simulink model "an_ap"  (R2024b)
settings: Solver=ode45  StartTime=0.0  StopTime=50  MaxStep=.1  RelTol=1e-3  AbsTol=1e-3  EnableMultiTasking=on
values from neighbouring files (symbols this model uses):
  den = 1    [ass_appr.m]    (also in simplify.m = a(find(a):max(size(a))); ass_sis.m; ass1_sis.m; myfbode.m = b)
  den_appr = 1    [ass_appr.m]    (also in ass_sis.m)
  num = b(find(b):max(size(b)))    [simplify.m]    (also in ass_sis.m = 0; ass1_sis.m = 0; myfbode.m = a; mynyq.m = a)
  num_appr = 0    [ass_appr.m]
  T = 0; end    [ass_appr.m]    (also in ass_sis.m = 0; ass1_sis.m = 0; myfbode.m = rit)
  T_appr = 0    [ass_appr.m]    (also in ass_sis.m = 0; end)

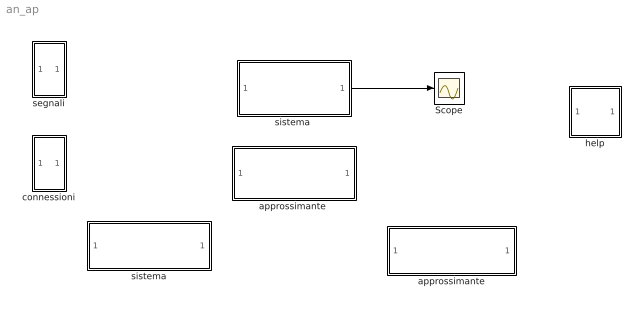
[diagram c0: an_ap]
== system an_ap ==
  Scope : Scope
  approssimante : Subsystem
  "approssimante " : Subsystem
  connessioni : Subsystem
  help : Subsystem
  segnali : Subsystem
  sistema : Subsystem
  "sistema " : Subsystem
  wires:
  "sistema "/1(out_1) -> Scope/1

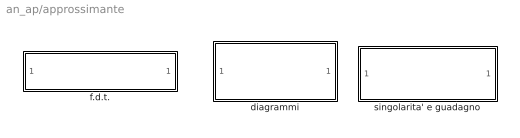
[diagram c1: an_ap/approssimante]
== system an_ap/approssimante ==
  diagrammi : Subsystem
  f.d.t. : Subsystem  mask(assegnamento f.d.t.){}
  singolarita' e guadagno : Subsystem  mask(singolarita' della f.d.t.){}

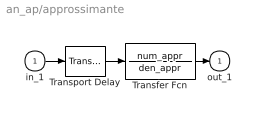
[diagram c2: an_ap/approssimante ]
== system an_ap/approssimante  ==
  in_1 : Inport
  Transfer Fcn : TransferFcn  Numerator=num_appr  Denominator=den_appr
  Transport Delay : TransportDelay  DelayTime=T_appr
  out_1 : Outport  VectorParamsAs1DForOutWhenUnconnected=off
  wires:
  Transport Delay/1 -> Transfer Fcn/1
  in_1/1 -> Transport Delay/1
  Transfer Fcn/1 -> out_1/1

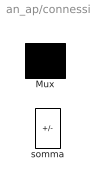
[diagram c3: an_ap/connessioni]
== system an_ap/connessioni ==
  Mux : Mux  Inputs=2
  somma : Sum  Inputs=+-  InputSameDT=on  SaturateOnIntegerOverflow=on

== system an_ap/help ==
  note: - il calcolo delle singolarità (poli e zeri), del guadagno e del ritardo della f.d.t.
  note: - l'inserimento della funzione di trasferimento
  note: - l'ottenimento dei diagrammi di Bode e di Nyquist
  note: i blocchi con l'ombreggiatura consentono

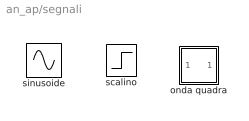
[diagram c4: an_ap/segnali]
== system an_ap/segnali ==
  onda quadra : Subsystem  mask(Pulse Generator){Ts=2, du=1, ht=1, stt=0}
      mask prompts: Ts "Pulse period (secs):"; du "Pulse width:"; ht "Pulse height:"; stt "Pulse start time:"
      mask help: Pulse Generator.
      mask init:
      | ini=ones(length(ht),1); st1=rem(stt,Ts); st2=rem(stt+du,Ts);if(Ts<=1.2*du),ini=zeros(length(ht),1);end;
  scalino : Step  Time=0
  sinusoide : Sin

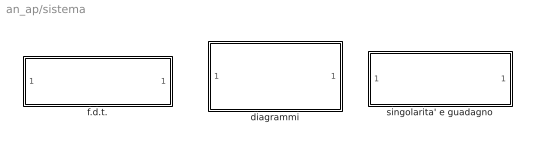
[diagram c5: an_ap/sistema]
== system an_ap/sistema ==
  diagrammi : Subsystem
  f.d.t. : Subsystem  mask(assegnamento f.d.t.){}
  singolarita' e guadagno : Subsystem  mask(singolarita' della f.d.t.){}

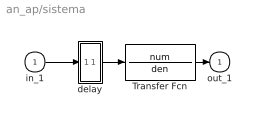
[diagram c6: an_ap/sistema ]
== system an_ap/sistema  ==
  in_1 : Inport
  Transfer Fcn : TransferFcn  Numerator=num  Denominator=den
  delay : Subsystem
  out_1 : Outport  VectorParamsAs1DForOutWhenUnconnected=off
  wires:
  delay/1(out_1) -> Transfer Fcn/1
  in_1/1 -> delay/1(in_1)
  Transfer Fcn/1 -> out_1/1

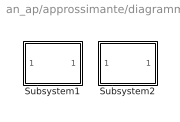
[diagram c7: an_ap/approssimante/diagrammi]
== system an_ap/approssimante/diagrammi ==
  Subsystem1 : Subsystem
  Subsystem2 : Subsystem

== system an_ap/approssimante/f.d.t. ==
  note: assegna

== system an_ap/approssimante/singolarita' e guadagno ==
  note: assegna

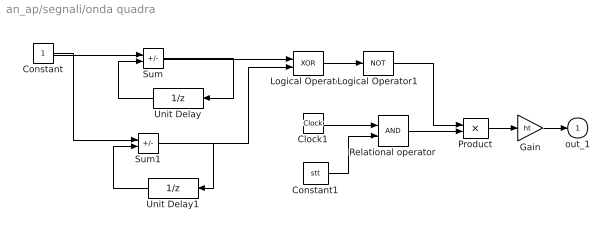
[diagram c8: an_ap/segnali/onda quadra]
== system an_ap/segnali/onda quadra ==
  Clock1 : Clock
  Constant : Constant
  Constant1 : Constant  Value=stt
  Gain : Gain  Gain=ht  SaturateOnIntegerOverflow=on
  Logical Operator : Logic  Operator=XOR
  Logical Operator1 : Logic  Operator=NOT  Inputs=1
  Product : Product  InputSameDT=on  SaturateOnIntegerOverflow=on
  Relational operator : RelationalOperator
  Sum : Sum  Inputs=+-  InputSameDT=on  SaturateOnIntegerOverflow=on
  Sum1 : Sum  Inputs=+-  InputSameDT=on  SaturateOnIntegerOverflow=on
  Unit Delay : UnitDelay  SampleTime=[Ts,st1]  HasFrameUpgradeWarning=on
  Unit Delay1 : UnitDelay  InitialCondition=ini  SampleTime=[Ts,st2]  HasFrameUpgradeWarning=on
  out_1 : Outport  VectorParamsAs1DForOutWhenUnconnected=off
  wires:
  Logical Operator1/1 -> Product/1
  Logical Operator/1 -> Logical Operator1/1
  Constant1/1 -> Relational operator/2
  Gain/1 -> out_1/1
  Product/1 -> Gain/1
  Relational operator/1 -> Product/2
  Clock1/1 -> Relational operator/1
  Unit Delay/1 -> Sum/2
  Unit Delay1/1 -> Sum1/2
  Constant/1 -> Sum/1, Sum1/1
  Sum/1 -> Unit Delay/1, Logical Operator/1
  Sum1/1 -> Unit Delay1/1, Logical Operator/2

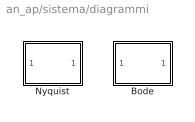
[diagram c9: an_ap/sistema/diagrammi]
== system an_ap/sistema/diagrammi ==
  Bode : Subsystem
  Nyquist : Subsystem

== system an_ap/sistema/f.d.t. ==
  note: assegna

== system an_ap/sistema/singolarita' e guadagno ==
  note: assegna

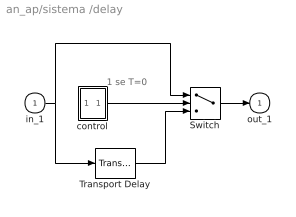
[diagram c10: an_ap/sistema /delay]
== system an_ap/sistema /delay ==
  note: 1 se T=0
  in_1 : Inport
  Switch : Switch  Threshold=.5
  Transport Delay : TransportDelay  DelayTime=T
  control : Subsystem
  out_1 : Outport  VectorParamsAs1DForOutWhenUnconnected=off
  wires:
  Transport Delay/1 -> Switch/3
  in_1/1 -> Switch/1, Transport Delay/1
  Switch/1 -> out_1/1
  control/1(out_1) -> Switch/2

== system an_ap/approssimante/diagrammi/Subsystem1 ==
  note: bode

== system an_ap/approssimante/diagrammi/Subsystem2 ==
  note: bode

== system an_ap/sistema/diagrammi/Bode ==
  note: bode

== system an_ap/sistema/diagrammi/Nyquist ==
  note: nyquist

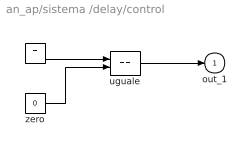
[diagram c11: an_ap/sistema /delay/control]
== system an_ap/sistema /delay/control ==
  T : Constant  Value=T
  uguale : RelationalOperator  Operator===
  zero : Constant  Value=0
  out_1 : Outport  VectorParamsAs1DForOutWhenUnconnected=off
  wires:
  zero/1 -> uguale/2
  T/1 -> uguale/1
  uguale/1 -> out_1/1
